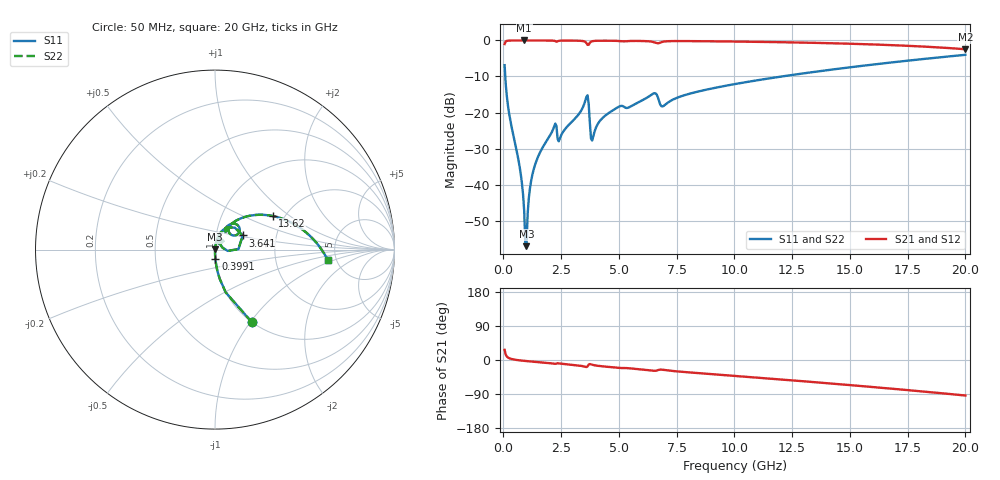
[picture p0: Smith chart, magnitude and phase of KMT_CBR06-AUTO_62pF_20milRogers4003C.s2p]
! Data measured by Modelithics Inc. support@modelithics.com 813-866-6335
! KEMET CBR06-AUTO 62pF, Pad Width= 0.851mm, Pad Length= 0.64mm, Pad Gap= 0.62mm, 20mil Rogers 4003C substrate Data, January 2022
# hz S ma R 50
! 2 Port Network Data from SP1.SP block
! freq  magS11  angS11  magS21  angS21  magS12  angS12  magS22  angS22
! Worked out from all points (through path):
!   401 points, 50 MHz to 20 GHz, reference 50 ohm
!   highest |S21| = 0.00 dB at 897.9 MHz (marker M1); lowest = -2.4 dB at 20 GHz (marker M2)
!   group delay of S21, straight-line fit = 13.1 ps
!   lowest |S11| = -57.1 dB at 997.6 MHz (marker M3), VSWR 1.00, Z = 50.1 + j0.128 ohm
!   |S11| at or under -10 dB: 79.31 MHz to 12.05 GHz (11.97 GHz wide, 197 % of centre)
!   |S22| runs from -57.1 to -4.0 dB; largest |S21 - S12| = 0
!   S11 on the Smith chart (normalised r, x): 50 MHz: 1.00, -1.02; 399.1 MHz: 1.00, -0.11; 3.641 GHz: 1.35, +0.22; 13.62 GHz: 1.74, +0.76; 20 GHz: 4.25, -0.85
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5e7  0.454 -63.1  0.8907 26.9  0.8907 26.9  0.454 -63.1
3.99125e8  0.05329 -87.7  0.9982 1.9  0.9982 1.9  0.05329 -87.7
7.4825e8  0.01409 -89.5  0.9994 -1.3  0.9994 -1.3  0.01409 -89.5
8.97875e8  0.004326 -85.9  0.9995 -2.3  0.9995 -2.3  0.004326 -85.9
9.97625e8  0.001401 66.1  0.9995 -2.9  0.9995 -2.9  0.001401 66.1
1.247e9  0.0135 83.3  0.9993 -4.2  0.9993 -4.2  0.0135 83.3
1.596125e9  0.02852 82.5  0.9988 -6.1  0.9988 -6.1  0.02852 82.5
2.194625e9  0.06371 72.5  0.9893 -9.7  0.9893 -9.7  0.06371 72.5
2.444e9  0.04391 71.4  0.9919 -9.3  0.9919 -9.3  0.04391 71.4
3.391625e9  0.1102 69.6  0.9849 -15.7  0.9849 -15.7  0.1102 69.6
3.641e9  0.1735 27.1  0.868 -17.1  0.868 -17.1  0.1735 27.1
3.890375e9  0.04696 56.0  0.9823 -13.3  0.9823 -13.3  0.04696 56.0
4.2395e9  0.0809 70.2  0.9918 -16.4  0.9918 -16.4  0.0809 70.2
4.93775e9  0.1176 65.7  0.9851 -20.4  0.9851 -20.4  0.1176 65.7
6.483875e9  0.1829 51.5  0.9511 -28.3  0.9511 -28.3  0.1829 51.5
6.73325e9  0.145 34.0  0.919 -25.9  0.919 -25.9  0.145 34.0
6.93275e9  0.1234 50.3  0.9634 -26.1  0.9634 -26.1  0.1234 50.3
1.0025e10  0.2484 47.3  0.9654 -42.0  0.9654 -42.0  0.2484 47.3
1.336662e10  0.3629 31.4  0.9276 -58.0  0.9276 -58.0  0.3629 31.4
1.3616e10  0.372 30.2  0.9239 -59.2  0.9239 -59.2  0.372 30.2
1.670825e10  0.4915 14.1  0.8634 -75.1  0.8634 -75.1  0.4915 14.1
2e10  0.6317 -5.4  0.7554 -93.7  0.7554 -93.7  0.6317 -5.4
